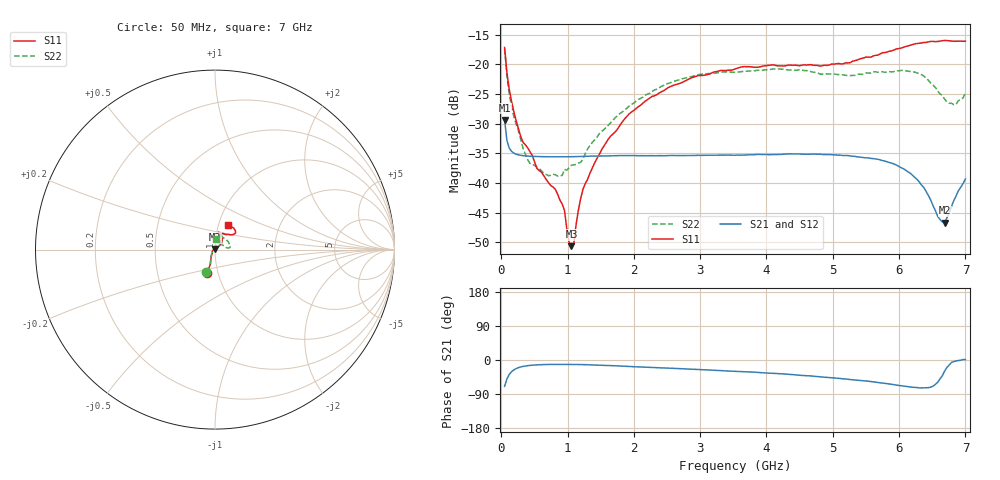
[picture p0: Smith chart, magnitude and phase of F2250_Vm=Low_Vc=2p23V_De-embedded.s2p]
! Integrated Device Technology
! Corporate Headquarters
! 6024 Silver Creek Valley Road
! San Jose, CA 95138  USA
! Phone:  1-408-284-8200
! Toll Free:  1-800-223-1366
! Webpage:  http://www.idt.com/
! Timing and RF Division
! 515 Groton Road, Suite 102
! Westford, MA 01886-6024
! Device:  F2250
! Description: Voltage Variable RF Attenuator
! Frequency:  50.0 -  6000.00 MHz
! Package:  3x3 mm Thin QFN Plastic Package: 16 pin
! Ports:  2 RF, 3 DC
!  Pin  1  = GND
!  Pin  2  = NC
!  Pin  3  = RF1  = Port 1
!  Pin  4  = NC
!  Pin  5  = GND
!  Pin  6  = GND
!  Pin  7  = GND
!  Pin  8  = GND
!  Pin  9  = NC
!  Pin 10  = RF2  = Port 2
!  Pin 11  = NC
!  Pin 12  = GND
!  Pin 13  = GND
!  Pin 14  = VCNTRL
!  Pin 15  = VDD
!  Pin 16  = VMODE
! Vcntrl:  2.230 Volts
! Vmode:  +0.000 Volts
! Vdd:  +3.30  Volts
! Current:  1.178 mA
! Data:  The device was measured on a the F2250 evaluation board which has
!  individual transmission lines to the RF pins.  Data was collected
!  using a calibrated network analyzer.  The evaluation board was
!  de-embedded using a TRL calibration technique.
!  The reference plane is the edge of the package pin.
! Misc:  SN 10
!  Action Tracker AT0258
! Date Measured:  2014-11-26
! Date:  2015-10-15  MJV
! Note:
!  Integrated Device Technology supplies this data as a sample of measured
!  data at the package pin for this product.  Your particular data for this
!  product may vary.
!  Data was taken at 25 degrees C.
!  Integrated Device Technology reserves the right to change this data at anytime.
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# GHz S dB R 50
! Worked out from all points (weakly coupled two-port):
!   201 points, 50 MHz to 7 GHz, reference 50 ohm
!   highest |S21| = -29.39 dB at 50 MHz (marker M1); lowest = -46.7 dB at 6.687 GHz (marker M2)
!   lowest |S11| = -50.7 dB at 1.058 GHz (marker M3), VSWR 1.01, Z = 49.8 + j0.243 ohm
!   |S11| at or under -10 dB: start of sweep to end of sweep
!   |S22| runs from -38.9 to -17.4 dB; largest |S21 - S12| = 6.1e-05
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0.05  -17.18 -108.6  -29.39 -69.5  -29.39 -69.5  -17.37 -110.6
0.08475  -21.44 -107.4  -32.87 -50.1  -32.87 -50.1  -21.89 -109.1
0.15425  -26.23 -116.6  -34.69 -31.0  -34.69 -31.0  -27.09 -120.4
0.29325  -32.20 -127.8  -35.36 -18.4  -35.36 -18.4  -32.67 -133.9
0.3975  -34.07 -141.8  -35.49 -15.0  -35.48 -15.0  -36.09 -157.6
0.71025  -39.95 -168.6  -35.60 -11.8  -35.60 -11.7  -38.79 153.9
0.91875  -43.56 158.0  -35.61 -11.6  -35.61 -11.6  -38.74 127.6
0.9535  -44.68 169.9  -35.61 -11.5  -35.61 -11.6  -37.73 125.9
1.023  -50.02 144.0  -35.60 -11.6  -35.60 -11.6  -37.44 109.1
1.05775  -50.67 123.7  -35.60 -11.7  -35.60 -11.7  -37.02 103.9
1.0925  -50.39 89.8  -35.59 -11.7  -35.58 -11.7  -36.97 98.9
1.162  -44.63 56.5  -35.57 -11.9  -35.56 -11.9  -36.66 87.9
1.2315  -41.08 44.3  -35.54 -12.2  -35.53 -12.2  -36.04 78.4
1.6485  -32.12 41.9  -35.45 -14.7  -35.45 -14.7  -29.88 60.8
2.37825  -24.87 47.3  -35.41 -20.4  -35.41 -20.4  -24.03 55.0
3.525  -20.80 72.5  -35.34 -29.7  -35.34 -29.7  -21.35 73.8
4.7065  -20.17 72.4  -35.14 -42.8  -35.14 -42.7  -21.34 71.8
5.85325  -17.82 40.5  -36.57 -63.4  -36.57 -63.4  -21.25 22.0
6.27025  -16.51 40.1  -39.40 -72.7  -39.40 -72.7  -21.46 8.6
6.68725  -15.99 48.8  -46.72 -29.1  -46.68 -28.8  -25.87 27.5
6.861  -16.12 55.1  -42.17 -2.3  -42.11 -2.2  -26.74 58.0
7  -16.12 63.3  -39.34 1.1  -39.30 1.0  -24.82 83.7
